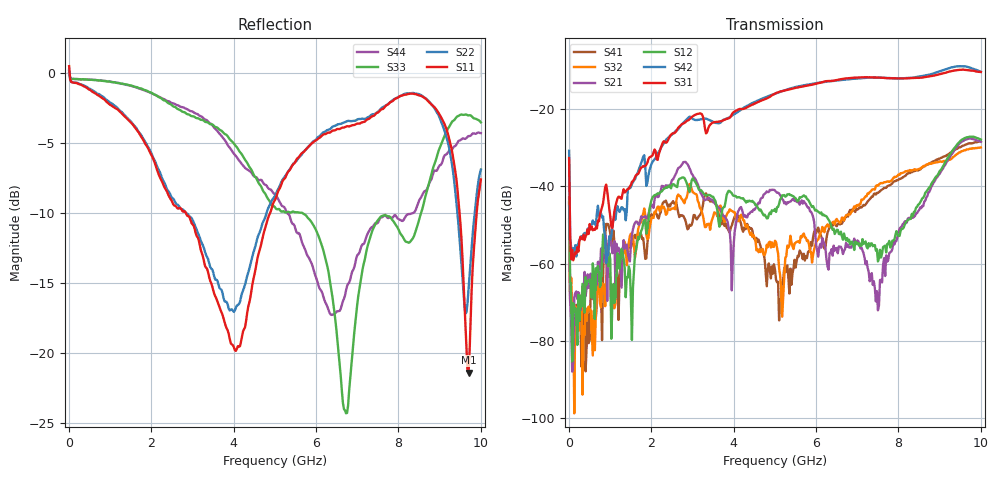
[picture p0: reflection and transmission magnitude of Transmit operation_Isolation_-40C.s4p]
! Device:  ADRF5545A
! Description: Dual-Channel, Receiver Front End
! Frequency:  2.4 -  4.2 GHz
! Ports:
!	ANT-CHA	= Port 1
!	ANT-CHB	= Port 2
!  TXOUT-CHA = Port 3
!	TXOUT-CHB = Port 4
! VDD1-CHA, VDD1-CHB, VDD2-CHA, VDD2-CHB, and SWVDD-CHAB = 5 V
! SWCTRL-CHAB = 0 V,  PD-CHAB = 0 V,BP-CHA=BP-CHB=0V
! Temp=-40C
! Data:  Data was collected using a calibrated 4 port network analyzer and de-embedded using AtaiTec's In Situ De-Embedding.
! Note:  Analog Devices supplies this data as a sample of measured data
!  for this product.  Your particular data for this product may vary.
!  Data was taken at -40 degrees C.
!  Analog Devices reserves the right to change this data at anytime.
!Correction: S11(Full 4 Port(1,2,3,4))
!S12(Full 4 Port(1,2,3,4))
!S13(Full 4 Port(1,2,3,4))
!S14(Full 4 Port(1,2,3,4))
!S21(Full 4 Port(1,2,3,4))
!S22(Full 4 Port(1,2,3,4))
!S23(Full 4 Port(1,2,3,4))
!S24(Full 4 Port(1,2,3,4))
!S31(Full 4 Port(1,2,3,4))
!S32(Full 4 Port(1,2,3,4))
!S33(Full 4 Port(1,2,3,4))
!S34(Full 4 Port(1,2,3,4))
!S41(Full 4 Port(1,2,3,4))
!S42(Full 4 Port(1,2,3,4))
!S43(Full 4 Port(1,2,3,4))
!S44(Full 4 Port(1,2,3,4))
!S4P File: Measurements: <S11,S12,S13,S14>,
!<S21,S22,S23,S24>,
!<S31,S32,S33,S34>,
!<S41,S42,S43,S44>:
# Hz S  dB  R 50
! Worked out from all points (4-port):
!   401 points, 10 MHz to 10 GHz, reference 50 ohm
!   strongest paths, dB at 10 MHz, 2.507 GHz, 5.005 GHz, 7.503 GHz, 10 GHz:
!     S31: -32.6, -26.4, -16.0, -11.8, -10.4
!     S42: -30.8, -26.6, -16.0, -11.8, -10.3
!     S12: -44.1, -39.6, -45.8, -59.4, -27.9
!     S21: -44.5, -38.3, -41.1, -72.1, -28.4
!     S32: -42.9, -45.7, -54.1, -39.8, -29.9
!     S41: -48.6, -44.2, -61.6, -41.7, -28.3
!   lowest |S11| = -21.4 dB at 9.7 GHz (marker M1), VSWR 1.19, Z = 43 + j3.72 ohm
!   |S11| at or under -10 dB: 2.843 GHz to 4.884 GHz (2.041 GHz wide, 52.8 % of centre); 9.483 GHz to 9.897 GHz (414.4 MHz wide, 4.28 % of centre)
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1e7  0.49 -20.3  -44.07 85.9  -36.02 26.9  -43.89 -26.7
     -44.45 -129.1  0.23 -19.6  -46.40 -116.3  -31.25 48.4
     -32.63 2.1  -42.90 -149.4  0.13 -10.8  -44.63 -110.8
     -48.57 -19.1  -30.77 70.9  -54.85 81.1  0.00 -9.3
3.84625e8  -0.96 -38.0  -72.71 76.1  -53.93 61.8  -71.45 3.7
           -62.13 66.3  -0.91 -38.3  -84.84 -82.4  -53.10 61.5
           -53.90 60.7  -78.46 111.4  -0.45 -18.0  -71.57 -26.6
           -67.39 48.9  -52.04 57.3  -76.25 -126.6  -0.45 -16.6
2.95705e9  -10.49 67.5  -40.18 58.1  -27.69 84.3  -64.69 30.7
           -35.90 10.4  -10.28 67.0  -64.48 88.0  -27.98 86.7
           -22.35 81.0  -39.55 76.3  -3.04 -131.9  -75.80 110.1
           -50.21 86.2  -21.99 78.1  -86.02 -127.9  -2.71 -120.5
5.2048e9  -7.63 41.9  -42.31 -35.0  -15.11 6.6  -66.25 91.6
          -43.56 -62.9  -7.54 36.5  -58.61 32.5  -14.92 12.0
          -15.29 9.6  -68.15 136.9  -9.86 103.4  -78.49 -16.4
          -63.94 68.8  -15.24 14.2  -71.29 143.2  -9.53 125.1
7.477525e9  -2.85 34.3  -56.23 117.2  -11.93 -84.0  -42.03 -98.1
            -67.13 107.1  -2.81 24.4  -43.09 -114.3  -11.99 -76.9
            -11.81 -83.8  -39.73 -109.4  -10.60 -98.0  -31.99 43.3
            -41.69 -102.3  -11.82 -76.3  -32.41 43.0  -10.74 -67.4
9.7003e9  -21.38 149.8  -27.22 -138.7  -9.91 178.0  -28.90 43.7
          -27.63 -145.6  -15.44 147.1  -31.44 19.4  -9.04 -177.5
          -9.92 177.4  -30.39 25.7  -3.02 161.2  -31.04 -178.8
          -28.86 41.1  -9.13 -178.5  -31.09 178.2  -4.50 -169.5
1e10  -7.59 -160.3  -27.87 168.8  -10.35 151.2  -28.24 4.5
      -28.45 162.1  -6.89 169.2  -31.14 -17.0  -10.21 154.2
      -10.37 150.5  -29.91 -11.5  -3.52 170.6  -29.21 164.2
      -28.34 1.3  -10.33 153.6  -29.41 160.4  -4.28 -161.8
